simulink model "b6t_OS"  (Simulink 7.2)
settings: Solver=ode3  SolverMode=SingleTasking  StartTime=0.0  StopTime=0.2  FixedStep=10e-6  MaxStep=1e-5  RelTol=1e-4  AbsTol=1e-4

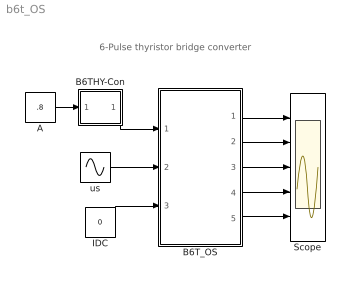
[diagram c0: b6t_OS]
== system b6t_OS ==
  note: 6-Pulse thyristor bridge converter
  A : Constant  Value=.8
  B6THY-Con : Subsystem  mask(B6THY-Con){F=50, PH=60, TD=1e-3}
      mask prompts: F "Frequency"; PH "Phase Angle (Degree)"; TD "Puls Duration"
      mask help: Control of one Thyristor in a line commutated Converter circuit
      mask init:
      | x=0:pi/20:2*pi;
      | y=cos(x);
  B6T_OS : Subsystem  mask{LS=1e-4, LD=1e-3, ILD0=200, C=2e-3, VC0=500, RL=2}
      mask prompts: LS "Source Inductance"; LD "DC Inductance LD"; ILD0 "Initial current ILD0"; C "Load Cap"; VC0 "Initial Cap Voltage"; RL "Load Resistance"
      mask help: 6-Pulse Thyristor Bridge Converter Input Vector u: u[0]= H1.gate u[1]= H2.gate u[2]= H3.gate u[3]= H4.gate u[4]= H5.gate u[5]= H6.gate u[6]= Vs1.v u[7]= Vs2.v u[8]= Vs3.v u[9]= IDC.i Output Vector y: y[0]= T11.I y[1]= T11.V y[2]= Lc1.I y[3]= Lc2.I y[4]= Lc3.I y[5]= Ld.I y[6]= VDC.V y[7]= VC.V Parameter Vector p: p[0]= Lc.L p[1]= Ld.L p[2]= Ld.IL0 p[3]= C1.C p[4]= C1.vC0 p[5]= R1.r You can pause the simulation during running, change the Parameters you want and continue the Simulation
  IDC : Constant  Value=0
  Scope : Scope  NumInputPorts=5
  us : Sin  Amplitude=230*sqrt(2)  Frequency=2*pi*50  Phase="[0,  -2*pi/3,  -4*pi/3]"  SampleTime=0
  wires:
  A/1 -> B6THY-Con/1(In1)
  B6THY-Con/1(Out1) -> B6T_OS/1(SWs)
  us/1 -> B6T_OS/2(vS)
  IDC/1 -> B6T_OS/3(iDC)
  B6T_OS/1(iT1,vT1) -> Scope/1
  B6T_OS/2("iLc1, iLc2, iLc3") -> Scope/2
  B6T_OS/3(iDC1) -> Scope/3
  B6T_OS/4(vDC) -> Scope/4
  B6T_OS/5(vC) -> Scope/5

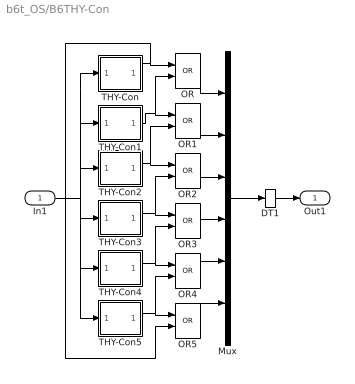
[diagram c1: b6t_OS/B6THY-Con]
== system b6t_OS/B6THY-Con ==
  In1 : Inport  OutDataType=sfix(16)  OutScaling=2^0
  DT1 : DataTypeConversion
  Mux : Mux  Inputs=6
  OR{,1..5} (6 alike) : Logic  Operator=OR
  THY-Con : Subsystem  mask(THY-Con){F=F, PH=PH, TD=TD}
      mask prompts: F "Frequency"; PH "Phase Angle (Degree)"; TD "Puls Duration"
      mask init:
      | x=0:pi/20:2*pi;
      | y=cos(x);
  THY-Con1 : Subsystem  mask(THY-Con){F=F, PH=PH-60, TD=TD}
      mask prompts: F "Frequency"; PH "Phase Angle (Degree)"; TD "Puls Duration"
      mask init:
      | x=0:pi/20:2*pi;
      | y=cos(x);
  THY-Con2 : Subsystem  mask(THY-Con){F=F, PH=PH-120, TD=TD}
      mask prompts: F "Frequency"; PH "Phase Angle (Degree)"; TD "Puls Duration"
      mask init:
      | x=0:pi/20:2*pi;
      | y=cos(x);
  THY-Con3 : Subsystem  mask(THY-Con){F=F, PH=PH-180, TD=TD}
      mask prompts: F "Frequency"; PH "Phase Angle (Degree)"; TD "Puls Duration"
      mask init:
      | x=0:pi/20:2*pi;
      | y=cos(x);
  THY-Con4 : Subsystem  mask(THY-Con){F=F, PH=PH-240, TD=TD}
      mask prompts: F "Frequency"; PH "Phase Angle (Degree)"; TD "Puls Duration"
      mask init:
      | x=0:pi/20:2*pi;
      | y=cos(x);
  THY-Con5 : Subsystem  mask(THY-Con){F=F, PH=PH-300, TD=TD}
      mask prompts: F "Frequency"; PH "Phase Angle (Degree)"; TD "Puls Duration"
      mask init:
      | x=0:pi/20:2*pi;
      | y=cos(x);
  Out1 : Outport
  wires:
  DT1/1 -> Out1/1
  In1/1 -> THY-Con/1(In1), THY-Con1/1(In1), THY-Con2/1(In1), THY-Con3/1(In1), THY-Con5/1(In1), THY-Con4/1(In1)
  Mux/1 -> DT1/1
  THY-Con1/1(Out1) -> OR1/1, OR/2
  THY-Con2/1(Out1) -> OR2/1, OR1/2
  THY-Con3/1(Out1) -> OR3/1, OR2/2
  THY-Con4/1(Out1) -> OR4/1, OR3/2
  THY-Con5/1(Out1) -> OR5/1, OR4/2
  THY-Con/1(Out1) -> OR/1, OR5/2
  OR/1 -> Mux/1
  OR1/1 -> Mux/2
  OR2/1 -> Mux/3
  OR3/1 -> Mux/4
  OR4/1 -> Mux/5
  OR5/1 -> Mux/6

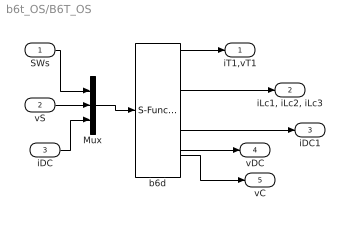
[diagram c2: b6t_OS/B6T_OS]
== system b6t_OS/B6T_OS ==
  SWs : Inport  OutDataType=sfix(16)  OutScaling=2^0
  vS : Inport  Port=2  OutDataType=sfix(16)  OutScaling=2^0
  iDC : Inport  Port=3  OutDataType=sfix(16)  OutScaling=2^0
  Mux : Mux  Inputs="[6 3  1]"
  b6d : S-Function  FunctionName=s_b6t_OS  Parameters="[ LS  LD ILD0 C  VC0 RL]"  EnableBusSupport=off
  iT1,vT1 : Outport  OutDataType=sfix(16)  OutScaling=2^0
  "iLc1, iLc2, iLc3" : Outport  Port=2  OutDataType=sfix(16)  OutScaling=2^0
  iDC1 : Outport  Port=3  OutDataType=sfix(16)  OutScaling=2^0
  vDC : Outport  Port=4  OutDataType=sfix(16)  OutScaling=2^0
  vC : Outport  Port=5  OutDataType=sfix(16)  OutScaling=2^0
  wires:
  b6d/4 -> vDC/1
  Mux/1 -> b6d/1
  iDC/1 -> Mux/3
  b6d/3 -> iDC1/1
  b6d/2 -> "iLc1, iLc2, iLc3"/1
  b6d/1 -> iT1,vT1/1
  vS/1 -> Mux/2
  SWs/1 -> Mux/1
  b6d/5 -> vC/1

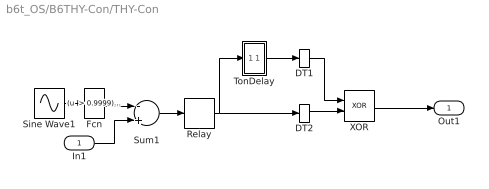
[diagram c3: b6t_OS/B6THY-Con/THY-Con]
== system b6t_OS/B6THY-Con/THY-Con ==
  In1 : Inport  OutDataType=sfix(16)  OutScaling=2^0
  DT1 : DataTypeConversion
  DT2 : DataTypeConversion
  Fcn : Fcn  Expr="(u  > 0.9999)*2 + (u<=0.9999)*u"
  Relay : Relay  OutDataType=sfix(16)  OutScaling=2^0
  Sine Wave1 : Sin  Frequency=F*2*pi  Phase=PH*pi/180  SampleTime=0
  Sum1 : Sum  Inputs=-+  OutDataType=sfix(16)  OutScaling=2^0
  TonDelay : Subsystem  mask(TonDelay){DT=TD}
      mask prompts: DT "Dead Time"
      mask help: Turn on dead time to protect against short circuit of the converter leg
  XOR : Logic  Operator=XOR
  Out1 : Outport
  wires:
  DT2/1 -> XOR/2
  DT1/1 -> XOR/1
  Fcn/1 -> Sum1/1
  Sine Wave1/1 -> Fcn/1
  XOR/1 -> Out1/1
  Relay/1 -> DT2/1, TonDelay/1(s1)
  TonDelay/1(s1d) -> DT1/1
  Sum1/1 -> Relay/1
  In1/1 -> Sum1/2

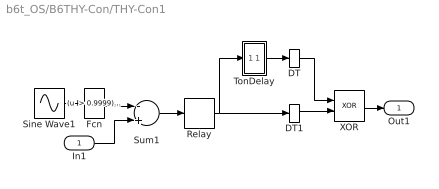
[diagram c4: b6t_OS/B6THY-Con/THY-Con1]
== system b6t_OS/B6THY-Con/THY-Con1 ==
  In1 : Inport  OutDataType=sfix(16)  OutScaling=2^0
  DT : DataTypeConversion
  DT1 : DataTypeConversion
  Fcn : Fcn  Expr="(u  > 0.9999)*2 + (u<=0.9999)*u"
  Relay : Relay  OutDataType=sfix(16)  OutScaling=2^0
  Sine Wave1 : Sin  Frequency=F*2*pi  Phase=PH*pi/180  SampleTime=0
  Sum1 : Sum  Inputs=-+  OutDataType=sfix(16)  OutScaling=2^0
  TonDelay : Subsystem  mask(TonDelay){DT=TD}
      mask prompts: DT "Dead Time"
      mask help: Turn on dead time to protect against short circuit of the converter leg
  XOR : Logic  Operator=XOR
  Out1 : Outport
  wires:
  DT1/1 -> XOR/2
  DT/1 -> XOR/1
  In1/1 -> Sum1/2
  Sum1/1 -> Relay/1
  TonDelay/1(s1d) -> DT/1
  Relay/1 -> DT1/1, TonDelay/1(s1)
  XOR/1 -> Out1/1
  Sine Wave1/1 -> Fcn/1
  Fcn/1 -> Sum1/1

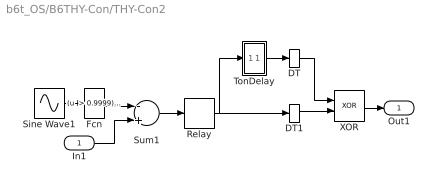
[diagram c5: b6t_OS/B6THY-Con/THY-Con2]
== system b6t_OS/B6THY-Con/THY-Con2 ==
  In1 : Inport  OutDataType=sfix(16)  OutScaling=2^0
  DT : DataTypeConversion
  DT1 : DataTypeConversion
  Fcn : Fcn  Expr="(u  > 0.9999)*2 + (u<=0.9999)*u"
  Relay : Relay  OutDataType=sfix(16)  OutScaling=2^0
  Sine Wave1 : Sin  Frequency=F*2*pi  Phase=PH*pi/180  SampleTime=0
  Sum1 : Sum  Inputs=-+  OutDataType=sfix(16)  OutScaling=2^0
  TonDelay : Subsystem  mask(TonDelay){DT=TD}
      mask prompts: DT "Dead Time"
      mask help: Turn on dead time to protect against short circuit of the converter leg
  XOR : Logic  Operator=XOR
  Out1 : Outport
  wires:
  DT1/1 -> XOR/2
  DT/1 -> XOR/1
  Fcn/1 -> Sum1/1
  Sine Wave1/1 -> Fcn/1
  XOR/1 -> Out1/1
  Relay/1 -> DT1/1, TonDelay/1(s1)
  TonDelay/1(s1d) -> DT/1
  Sum1/1 -> Relay/1
  In1/1 -> Sum1/2

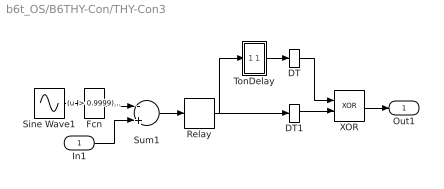
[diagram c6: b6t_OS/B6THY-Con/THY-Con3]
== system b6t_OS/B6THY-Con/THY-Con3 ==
  In1 : Inport  OutDataType=sfix(16)  OutScaling=2^0
  DT : DataTypeConversion
  DT1 : DataTypeConversion
  Fcn : Fcn  Expr="(u  > 0.9999)*2 + (u<=0.9999)*u"
  Relay : Relay  OutDataType=sfix(16)  OutScaling=2^0
  Sine Wave1 : Sin  Frequency=F*2*pi  Phase=PH*pi/180  SampleTime=0
  Sum1 : Sum  Inputs=-+  OutDataType=sfix(16)  OutScaling=2^0
  TonDelay : Subsystem  mask(TonDelay){DT=TD}
      mask prompts: DT "Dead Time"
      mask help: Turn on dead time to protect against short circuit of the converter leg
  XOR : Logic  Operator=XOR
  Out1 : Outport
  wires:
  DT1/1 -> XOR/2
  DT/1 -> XOR/1
  In1/1 -> Sum1/2
  Sum1/1 -> Relay/1
  TonDelay/1(s1d) -> DT/1
  Relay/1 -> DT1/1, TonDelay/1(s1)
  XOR/1 -> Out1/1
  Sine Wave1/1 -> Fcn/1
  Fcn/1 -> Sum1/1

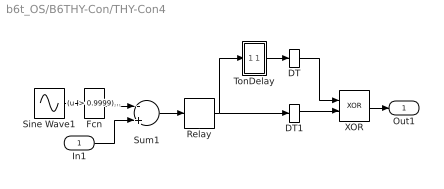
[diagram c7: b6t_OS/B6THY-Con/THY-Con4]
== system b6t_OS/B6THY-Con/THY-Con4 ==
  In1 : Inport  OutDataType=sfix(16)  OutScaling=2^0
  DT : DataTypeConversion
  DT1 : DataTypeConversion
  Fcn : Fcn  Expr="(u  > 0.9999)*2 + (u<=0.9999)*u"
  Relay : Relay  OutDataType=sfix(16)  OutScaling=2^0
  Sine Wave1 : Sin  Frequency=F*2*pi  Phase=PH*pi/180  SampleTime=0
  Sum1 : Sum  Inputs=-+  OutDataType=sfix(16)  OutScaling=2^0
  TonDelay : Subsystem  mask(TonDelay){DT=TD}
      mask prompts: DT "Dead Time"
      mask help: Turn on dead time to protect against short circuit of the converter leg
  XOR : Logic  Operator=XOR
  Out1 : Outport
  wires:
  DT1/1 -> XOR/2
  DT/1 -> XOR/1
  Fcn/1 -> Sum1/1
  Sine Wave1/1 -> Fcn/1
  XOR/1 -> Out1/1
  Relay/1 -> DT1/1, TonDelay/1(s1)
  TonDelay/1(s1d) -> DT/1
  Sum1/1 -> Relay/1
  In1/1 -> Sum1/2

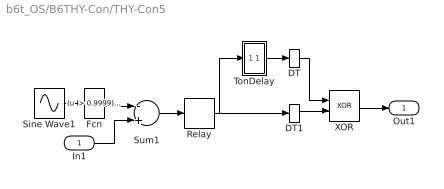
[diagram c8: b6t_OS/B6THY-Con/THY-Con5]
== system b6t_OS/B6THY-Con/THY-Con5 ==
  In1 : Inport  OutDataType=sfix(16)  OutScaling=2^0
  DT : DataTypeConversion
  DT1 : DataTypeConversion
  Fcn : Fcn  Expr="(u  > 0.9999)*2 + (u<=0.9999)*u"
  Relay : Relay  OutDataType=sfix(16)  OutScaling=2^0
  Sine Wave1 : Sin  Frequency=F*2*pi  Phase=PH*pi/180  SampleTime=0
  Sum1 : Sum  Inputs=-+  OutDataType=sfix(16)  OutScaling=2^0
  TonDelay : Subsystem  mask(TonDelay){DT=TD}
      mask prompts: DT "Dead Time"
      mask help: Turn on dead time to protect against short circuit of the converter leg
  XOR : Logic  Operator=XOR
  Out1 : Outport
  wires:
  DT1/1 -> XOR/2
  DT/1 -> XOR/1
  In1/1 -> Sum1/2
  Sum1/1 -> Relay/1
  TonDelay/1(s1d) -> DT/1
  Relay/1 -> DT1/1, TonDelay/1(s1)
  XOR/1 -> Out1/1
  Sine Wave1/1 -> Fcn/1
  Fcn/1 -> Sum1/1

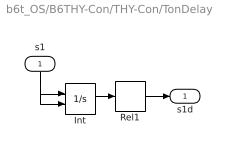
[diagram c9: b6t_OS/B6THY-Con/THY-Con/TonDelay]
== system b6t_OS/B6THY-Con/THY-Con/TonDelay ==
  s1 : Inport  Orientation=down  OutDataType=sfix(16)  OutScaling=2^0
  Int : Integrator  ExternalReset=falling
  Rel1 : Relay  OnSwitchValue=DT  OutDataType=sfix(16)  OutScaling=2^0
  s1d : Outport  InitialOutput=0
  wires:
  Rel1/1 -> s1d/1
  s1/1 -> Int/1, Int/2
  Int/1 -> Rel1/1

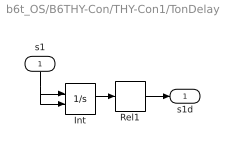
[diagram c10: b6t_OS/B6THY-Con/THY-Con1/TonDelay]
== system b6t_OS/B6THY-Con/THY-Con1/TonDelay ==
  s1 : Inport  Orientation=down  OutDataType=sfix(16)  OutScaling=2^0
  Int : Integrator  ExternalReset=falling
  Rel1 : Relay  OnSwitchValue=DT  OutDataType=sfix(16)  OutScaling=2^0
  s1d : Outport  InitialOutput=0
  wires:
  Rel1/1 -> s1d/1
  s1/1 -> Int/1, Int/2
  Int/1 -> Rel1/1

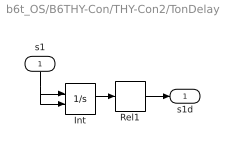
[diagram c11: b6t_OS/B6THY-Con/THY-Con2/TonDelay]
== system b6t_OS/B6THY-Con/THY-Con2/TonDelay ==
  s1 : Inport  Orientation=down  OutDataType=sfix(16)  OutScaling=2^0
  Int : Integrator  ExternalReset=falling
  Rel1 : Relay  OnSwitchValue=DT  OutDataType=sfix(16)  OutScaling=2^0
  s1d : Outport  InitialOutput=0
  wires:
  Rel1/1 -> s1d/1
  s1/1 -> Int/1, Int/2
  Int/1 -> Rel1/1

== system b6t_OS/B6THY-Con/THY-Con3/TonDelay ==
  s1 : Inport  Orientation=down  OutDataType=sfix(16)  OutScaling=2^0
  Int : Integrator  ExternalReset=falling
  Rel1 : Relay  OnSwitchValue=DT  OutDataType=sfix(16)  OutScaling=2^0
  s1d : Outport  InitialOutput=0
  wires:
  Rel1/1 -> s1d/1
  s1/1 -> Int/1, Int/2
  Int/1 -> Rel1/1

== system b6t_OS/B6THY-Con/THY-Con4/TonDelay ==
  s1 : Inport  Orientation=down  OutDataType=sfix(16)  OutScaling=2^0
  Int : Integrator  ExternalReset=falling
  Rel1 : Relay  OnSwitchValue=DT  OutDataType=sfix(16)  OutScaling=2^0
  s1d : Outport  InitialOutput=0
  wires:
  Rel1/1 -> s1d/1
  s1/1 -> Int/1, Int/2
  Int/1 -> Rel1/1

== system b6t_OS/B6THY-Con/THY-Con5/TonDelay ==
  s1 : Inport  Orientation=down  OutDataType=sfix(16)  OutScaling=2^0
  Int : Integrator  ExternalReset=falling
  Rel1 : Relay  OnSwitchValue=DT  OutDataType=sfix(16)  OutScaling=2^0
  s1d : Outport  InitialOutput=0
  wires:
  Rel1/1 -> s1d/1
  s1/1 -> Int/1, Int/2
  Int/1 -> Rel1/1
